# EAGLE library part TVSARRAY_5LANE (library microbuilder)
Voltage Transient Suppressor Array SOT363 SMF05C - 100W 5V: Digikey - SMF05CT1GOSCT-ND
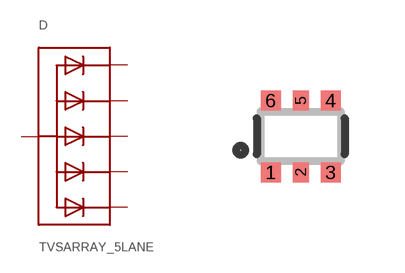
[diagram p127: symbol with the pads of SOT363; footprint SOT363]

Designator prefix D

## TVSARRAY_5LANE  [SOT363]
1  C1  pas
2  A  pas
3  C2  pas
4  C3  pas
5  C4  pas
6  C5  pas

## Footprint SOT363 (pad centres in mm)
Source: http://www.nxp.com/documents/data_sheet/2N7002PS.pdf
smd 0.5 x 0.5: 1 -0.75,-0.9; 3 0.75,-0.9; 4 0.75,0.9; 6 -0.75,0.9
smd 0.4 x 0.5: 2 0,-0.9; 5 0,0.9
